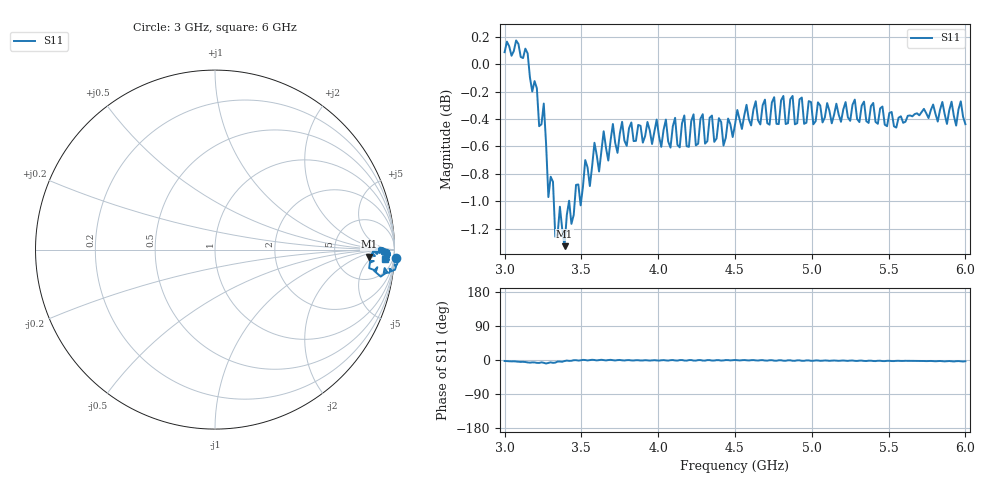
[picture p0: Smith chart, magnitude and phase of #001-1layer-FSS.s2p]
!  05/08/2025  15:20:16
! Ref Plane: 0.000 mm
# MHZ S MA R  50
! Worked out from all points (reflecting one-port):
!   201 points, 3 GHz to 6 GHz, reference 50 ohm
!   lowest |S11| = -1.3 dB at 3.39 GHz (marker M1), VSWR 13.11, Z = 600 - j182 ohm
!   phase of S11 starts at -3 deg and turns -1 deg over the sweep
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3000  1.01 -2.5
3135  1.013 -5.3
3210  0.9799 -7.5
3240  0.9507 -6.2
3255  0.9674 -7.4
3270  0.9353 -9.2
3285  0.8944 -7.6
3300  0.9098 -6.2
3330  0.8651 -6.9
3345  0.8666 -4.1
3375  0.8708 -4.7
3390  0.8583 -2.7
3525  0.9226 -0.0
3555  0.9027 -0.3
3585  0.9361 -0.0
3615  0.9138 -0.1
3645  0.9452 -0.2
3675  0.9222 -0.1
3750  0.9432 0.1
4125  0.9345 -1.6
4155  0.9515 -0.1
4245  0.9341 -1.6
4500  0.9504 0.1
4875  0.9736 -2.0
4890  0.9507 -2.1
5250  0.9535 -1.5
5625  0.9575 -2.2
6000  0.9508 -3.3
